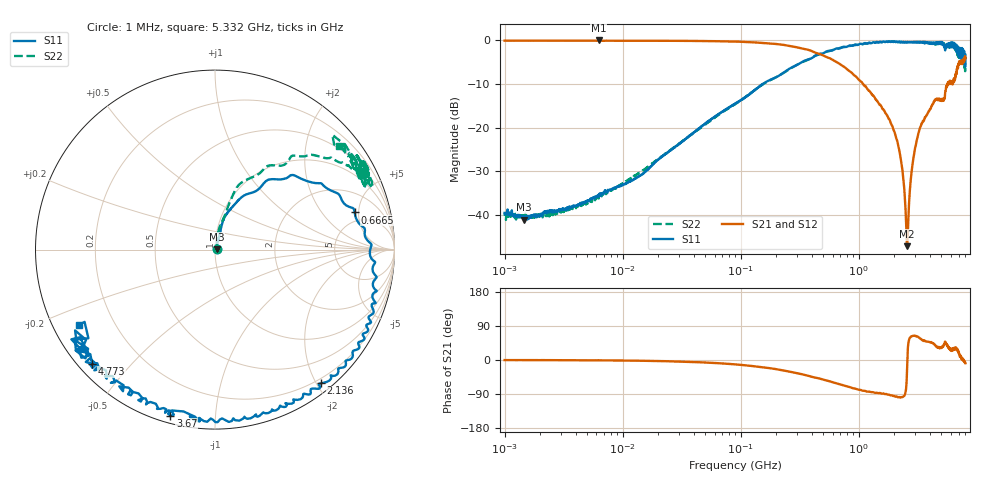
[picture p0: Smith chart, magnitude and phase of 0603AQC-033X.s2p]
!s-Parameter Generated by FASTRON Sdn. Bhd.
!FASTRON P/N : 0603AQC-033X
!Keysight Technologies: E5071C_MY46733604_B.14.02
!Date: Thu Jun 25 13:53:18 2026
!Version  :Rev00  Thu Jun 25 13:53:18 2026
!Data & Calibration Information:
!Freq  S11:SOLT2(ON)  S21:SOLT2(ON)  S12:SOLT2(ON)  S22:SOLT2(ON)
!PortZ  Port1:50+j0  Port2:50+j0
!When reading reference impedance value at option line is always used.
! Remarks : This data is being provided solely for informational purposes.
# Hz S dB R 50
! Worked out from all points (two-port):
!   1601 points, 1 MHz to 8 GHz, reference 50 ohm
!   highest |S21| = -0.04 dB at 6.268 MHz (marker M1); lowest = -47.1 dB at 2.56 GHz (marker M2)
!   |S21| within 3 dB of the highest: start of sweep to 450.2 MHz
!   lowest |S11| = -41.0 dB at 1.468 MHz (marker M3), VSWR 1.02, Z = 50.9 + j0.215 ohm
!   |S11| at or under -10 dB: start of sweep to 153.3 MHz
!   |S22| runs from -41.1 to -0.3 dB; largest |S21 - S12| = 0.026
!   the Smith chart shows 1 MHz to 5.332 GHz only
!   S11 on the Smith chart (normalised r, x): 1 MHz: 1.02, +0.00; 666.5 MHz: 3.82, +4.50; 2.136 GHz: 0.13, -2.06; 3.67 GHz: 0.03, -0.77; 4.773 GHz: 0.04, -0.39; 5.332 GHz: 0.08, -0.26
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1000000  -39.50 8.9  -0.09 -0.2  -0.09 -0.2  -40.20 10.9
1468277  -41.00 13.7  -0.09 -0.3  -0.10 -0.2  -40.00 9.0
4479405  -37.20 43.1  -0.10 -0.6  -0.08 -0.7  -37.90 48.0
6268472  -35.60 46.5  -0.04 -0.6  -0.21 -1.4  -36.20 55.6
2.00676e7  -27.30 69.2  -0.12 -2.8  -0.11 -2.7  -27.10 76.2
8.994653e7  -14.50 73.6  -0.30 -11.6  -0.30 -11.6  -14.60 74.4
2.06683e8  -8.23 55.9  -0.89 -25.0  -0.90 -25.0  -8.23 69.5
4.006501e8  -4.06 38.6  -2.47 -44.4  -2.47 -44.4  -3.96 50.4
6.665231e8  -1.88 14.9  -5.15 -62.7  -5.15 -62.8  -1.89 39.2
1.165105e9  -0.77 -15.5  -10.90 -83.1  -10.90 -83.2  -0.73 26.9
1.7949e9  -0.28 -37.5  -18.00 -91.3  -18.00 -91.4  -0.31 30.1
2.135779e9  -0.44 -51.6  -23.50 -98.2  -23.50 -98.3  -0.37 28.2
2.325502e9  -0.44 -57.8  -29.00 -98.1  -29.00 -98.2  -0.44 27.4
2.560258e9  -0.48 -65.2  -47.10 -30.3  -47.20 -31.2  -0.44 28.0
3.044443e9  -0.49 -80.0  -23.90 63.1  -23.90 63.1  -0.46 32.6
3.669656e9  -0.36 -105.0  -17.60 49.2  -17.50 49.1  -0.59 28.1
4.135839e9  -0.72 -121.0  -15.00 46.0  -15.00 45.7  -0.80 34.4
4.772513e9  -0.58 -137.0  -13.60 34.4  -13.60 34.2  -0.64 28.3
5.33235e9  -1.26 -151.0  -13.40 43.1  -13.40 42.8  -0.90 39.9
6.419251e9  -0.60 -169.0  -9.48 27.4  -9.47 27.0  -1.32 48.8
6.959019e9  -3.39 -171.0  -5.40 24.1  -5.37 23.4  -3.83 59.1
8e9  -3.33 145.0  -4.13 -8.8  -4.16 -9.4  -5.27 49.7
